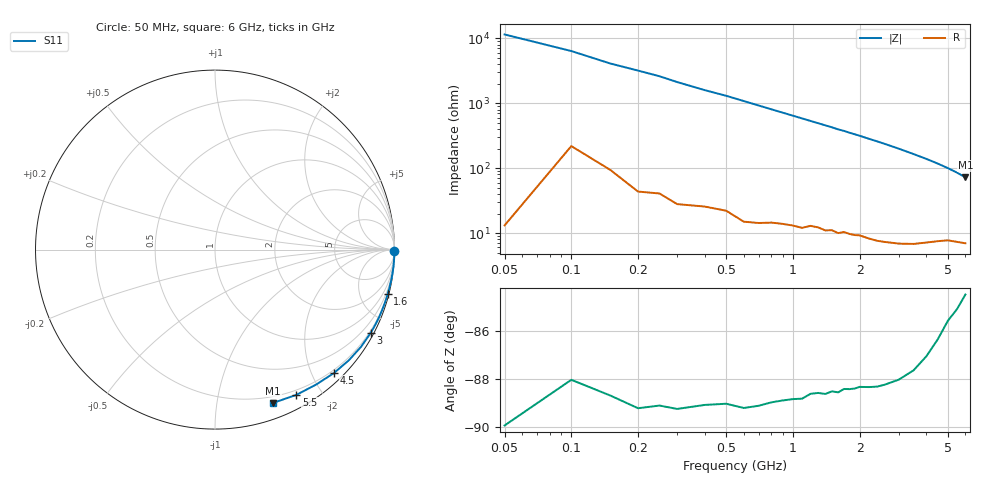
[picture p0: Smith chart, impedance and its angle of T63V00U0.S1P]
! SIEMENS Discrete & RF Semiconductors
! BAT62
! Si Schottky Diode in SOT143
! VR = 3 V
! S-Parameters:  February  1997
# GHz  S  MA  R  50
!  f  S11
! GHz  MAG  ANG
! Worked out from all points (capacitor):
!   34 points, 50 MHz to 6 GHz, reference 50 ohm
!   read as one part to ground: C = 259 fF near 50 MHz
!   lowest |Z| = 72.2 ohm at 6 GHz (marker M1)
!   S11 on the Smith chart (normalised r, x): 50 MHz: open; 1.6 GHz: 0.20, -7.91; 3 GHz: 0.14, -3.99; 4.5 GHz: 0.15, -2.35; 5.5 GHz: 0.15, -1.70; 6 GHz: 0.14, -1.44
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0.05  1 -0.5
0.1  0.9995 -0.9
0.15  0.9994 -1.4
0.25  0.9994 -2.2
0.3  0.9994 -2.7
0.4  0.999 -3.6
0.5  0.9987 -4.4
0.6  0.9987 -5.3
0.8  0.9978 -7.1
1.1  0.9965 -9.8
1.4  0.9948 -12.5
1.5  0.994 -13.4
1.6  0.9937 -14.4
1.7  0.9928 -15.2
1.8  0.9923 -16.2
1.9  0.9918 -17.1
2  0.991 -18.0
2.2  0.9901 -20.0
2.4  0.9891 -21.9
2.6  0.9876 -23.9
2.8  0.9858 -26.0
3  0.9839 -28.1
3.5  0.9774 -33.7
4  0.9677 -39.6
4.5  0.9551 -46.0
5  0.94 -53.0
5.5  0.9278 -60.7
6  0.9136 -69.3
